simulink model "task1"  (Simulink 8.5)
undefined symbols (not defined in the file): Double, F64, I32, Long
libraries: mathlib x13, matrixlib x9, arclib x6, genlib x2, modellib x1, execlib x1, speclib x1, langlib x1

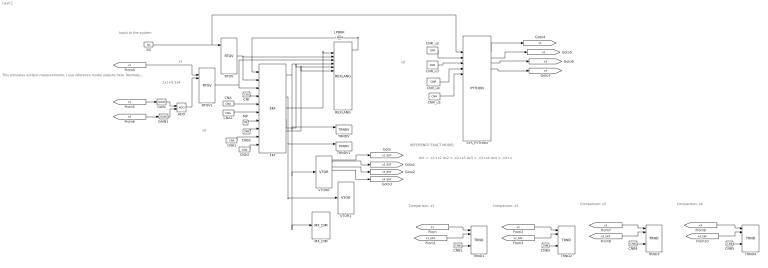
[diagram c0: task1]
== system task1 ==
  note: REFERENCE EXACT MODEL
  note: 2x1+0.5x4
  note: x1
  note: This emulates outtput measurements. I use reference model outputs here. Normaly, this would be taken from real measured data.
  note: Input to the system
  note: Comparison: x1
  note: Comparison: x2
  note: Comparison: x3
  note: Comparison: x4
  note: dx1 = -x1+x2 dx2 = -x2+x3 dx3 = -x3+x4 dx4 = -x4+u
  note: x0
  note: x0
  ADD : mathlib/ADD
  CNA : matrixlib/CNA  TRN=off  nmax=100  etype=8: Double  acn=[1 0 0 0; 0 1 0 0; 0 0 1 0; 0 0 0 1]
  CNA1 : matrixlib/CNA  TRN=off  nmax=100  etype=8: Double  acn=[0; 0; 0; 0]
  CNA2 : matrixlib/CNA  TRN=off  nmax=100  etype=8: Double  acn=[0.1 0; 0 .1]
  CNA3 : matrixlib/CNA  TRN=off  nmax=100  etype=8: Double  acn=[0.1 0 0 0; 0 0.1 0 0; 0 0 0.01 0; 0 0 0 0.01]
  CNB{1,3..5} (4 alike) : mathlib/CNB  YCN=on
  CNB2 : mathlib/CNB  YCN=off
  CNI : mathlib/CNI  icn=1  vtype=4: Long (I32)
  CNR_u{2..5} (4 alike) : mathlib/CNR  ycn=0
  EKF : modellib/EKF  nmax=100  solver=7: 4th order Runge-Kutha
  GAIN : mathlib/GAIN  k=2
  GAIN1 : mathlib/GAIN  k=0.5
  LPBRK : execlib/LPBRK  Orientation=left  RB=off
  MP : genlib/MP  BSTATE=off  pwidth=1  RPTF=off
  MX_DIM : matrixlib/MX_DIM
  REXLANG : speclib/REXLANG  tab_matlab=BASIC  srcname=test_lin.c  srctype=1: C-like  debug=3: Full check  stack=0  strs=0  p0=0  p1=0  p2=0  p3=0  p4=0  p5=0  p6=0  p7=0  p8=0  p9=0  p10=0  p11=0  p12=0  p13=0  p14=0  p15=0
  RTOV : matrixlib/RTOV  nmax=8  offset=0  n=2  etype=8: Double
  RTOV1 : matrixlib/RTOV  nmax=8  offset=0  n=2  etype=8: Double
  SG : genlib/SG  isig=1: SINE  amp=1  freq=1  phase=0  offset=0  ifrunit=1: Hz  iphunit=1: degrees
  SYS_PYTHON : langlib/PYTHON  srcname=sys.py  embedded=on
  TRND{1..4} (4 alike) : arclib/TRND  n=2  l=1000  btype=8: Double (F64)  ptype1=1: Store  ptype2=1: Store  ptype3=1: Store  ptype4=1: Store  pfac=1  afac=1  arc=0  id=0  title=Trend Title  timesrc=1: CORETIMER
  TRNDV : arclib/TRNDV  n=8  l=1000  btype=8: Double  pfac=1  afac=0  arc=0  id=1  Title=Trend Title  timesrc=1: CORETIMER
  TRNDV1 : arclib/TRNDV  n=8  l=1000  btype=8: Double  pfac=1  afac=0  arc=0  id=1  Title=Trend Title  timesrc=1: CORETIMER
  VTOR1 : matrixlib/VTOR  n=8  offset=0  etype=8: Double
  VTOR6 : matrixlib/VTOR  n=8  offset=0  etype=8: Double
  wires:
  ADD/1 -> RTOV1/3
  CNA/1 -> EKF/5
  CNA1/1 -> EKF/9
  CNA2/1 -> EKF/6
  CNA3/1 -> EKF/10
  CNB1/1 -> TRND1/5
  CNB2/1 -> EKF/8
  CNB3/1 -> TRND2/5
  CNB4/1 -> TRND3/5
  CNB5/1 -> TRND4/5
  CNI/1 -> EKF/4
  CNR_u2/1 -> SYS_PYTHON/4
  CNR_u3/1 -> SYS_PYTHON/5
  CNR_u4/1 -> SYS_PYTHON/6
  CNR_u5/1 -> SYS_PYTHON/7
  EKF/1 -> TRNDV/1, MX_DIM/1, VTOR6/1, REXLANG/6
  EKF/3 -> TRNDV1/1, VTOR1/1
  EKF/4 -> REXLANG/3
  EKF/5 -> REXLANG/7
  EKF/6 -> REXLANG/8
  [x1] -> TRND1/1
  [x1_EKF] -> TRND1/2
  [x4_EKF] -> TRND4/2
  [x2] -> TRND2/1
  [x2_EKF] -> TRND2/2
  [x1] -> RTOV1/2
  [x1] -> GAIN/1
  [x4] -> GAIN1/1
  [x3] -> TRND3/1
  [x3_EKF] -> TRND3/2
  [x4] -> TRND4/1
  GAIN/1 -> ADD/1
  GAIN1/1 -> ADD/2
  LPBRK/1 -> EKF/1
  MP/1 -> EKF/7
  REXLANG/2 -> LPBRK/1
  RTOV/1 -> EKF/2, REXLANG/4
  RTOV1/1 -> EKF/3, REXLANG/5
  SG/1 -> RTOV/2, SYS_PYTHON/3
  SYS_PYTHON/3 -> [x1]
  SYS_PYTHON/4 -> [x2]
  SYS_PYTHON/5 -> [x3]
  SYS_PYTHON/6 -> [x4]
  VTOR6/1 -> [x1_EKF]
  VTOR6/2 -> [x2_EKF]
  VTOR6/3 -> [x3_EKF]
  VTOR6/4 -> [x4_EKF]
